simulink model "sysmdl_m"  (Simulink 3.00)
settings: Solver=ode23s  SolverMode=SingleTasking  StartTime=0.0  StopTime=50.0  RelTol=1e-3  AbsTol=1e-6
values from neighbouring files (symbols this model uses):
  c = fminsearch('pdn_prf',k,options)    [optimise.m]    (also in optimise_new.m = fminsearch('pdn_prf_new',k,options))

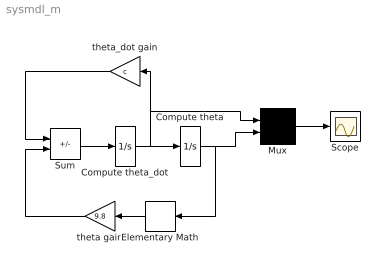
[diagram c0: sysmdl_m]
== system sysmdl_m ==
  Compute theta : Integrator  ExternalReset=none  InitialConditionSource=internal  InitialCondition=pi/3  LimitOutput=off  UpperSaturationLimit=inf  LowerSaturationLimit=-inf  ShowSaturationPort=off  ShowStatePort=off  AbsoluteTolerance=auto
  Compute theta_dot : Integrator  ExternalReset=none  InitialConditionSource=internal  InitialCondition=0  LimitOutput=off  UpperSaturationLimit=inf  LowerSaturationLimit=-inf  ShowSaturationPort=off  ShowStatePort=off  AbsoluteTolerance=auto
  Elementary Math : ElementaryMath  Orientation=left  Operator=sin
  Mux : Mux  Inputs=2
  Scope : Scope
  Sum : Sum  Inputs=--  SaturateOnIntegerOverflow=on
  theta gain : Gain  Orientation=left  Gain=9.8  SaturateOnIntegerOverflow=on
  theta_dot gain : Gain  Orientation=left  Gain=c  SaturateOnIntegerOverflow=on
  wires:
  Compute theta_dot/1 -> Compute theta/1, theta_dot gain/1, Mux/1
  Sum/1 -> Compute theta_dot/1
  theta_dot gain/1 -> Sum/1
  Mux/1 -> Scope/1
  Compute theta/1 -> Mux/2, Elementary Math/1
  Elementary Math/1 -> theta gain/1
  theta gain/1 -> Sum/2
